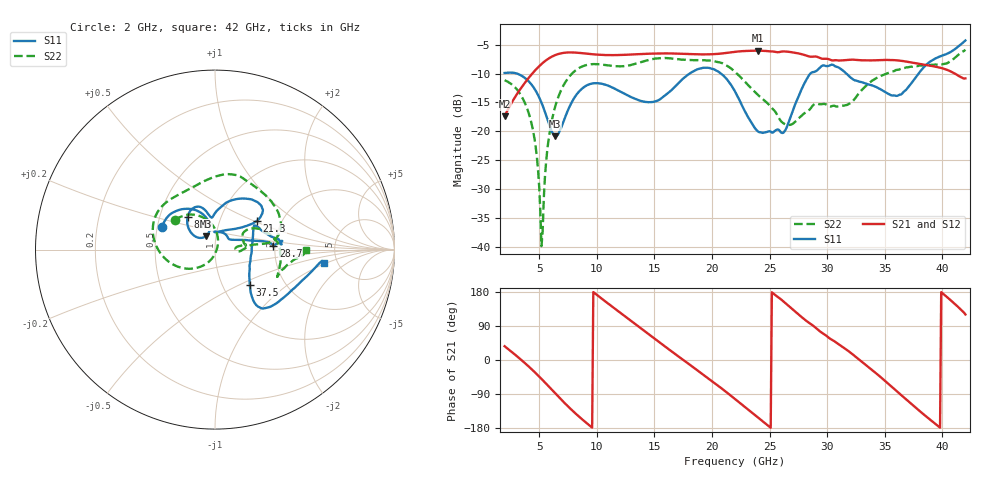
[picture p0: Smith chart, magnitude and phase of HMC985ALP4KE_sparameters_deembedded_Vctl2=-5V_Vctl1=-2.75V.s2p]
!s2p File: Measurements: S11, S21, S12, S22
# GHz S dB R 50.0
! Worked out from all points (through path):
!   401 points, 2 GHz to 42 GHz, reference 50 ohm
!   highest |S21| = -6.03 dB at 24 GHz (marker M1); lowest = -17.4 dB at 2 GHz (marker M2)
!   lowest |S11| = -20.9 dB at 6.4 GHz (marker M3), VSWR 1.20, Z = 44.7 + j6.77 ohm
!   |S11| at or under -10 dB: 3.095 GHz to 18.05 GHz (14.96 GHz wide, 141 % of centre); 20.79 GHz to 28.54 GHz (7.748 GHz wide, 31.4 % of centre); 31.67 GHz to 37.93 GHz (6.262 GHz wide, 18 % of centre)
!   |S22| runs from -39.9 to -5.9 dB; largest |S21 - S12| = 0.00055
!   S11 on the Smith chart (normalised r, x): 2 GHz: 0.53, +0.15; 8.8 GHz: 0.69, +0.27; 21.3 GHz: 1.50, +0.52; 28.7 GHz: 1.96, +0.10; 37.5 GHz: 1.34, -0.57; 42 GHz: 3.92, -0.95
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2  -9.89 157.1  -17.40 36.4  -17.41 36.4  -11.14 143.7
4.2  -11.57 121.0  -10.47 -20.1  -10.47 -20.1  -17.57 94.6
4.7  -12.97 111.9  -9.33 -34.6  -9.33 -34.6  -22.74 78.3
5.2  -15.03 104.5  -8.35 -49.8  -8.35 -49.8  -39.88 6.8
5.4  -16.06 102.8  -8.00 -56.0  -8.01 -56.0  -31.66 -92.8
5.8  -18.39 103.8  -7.41 -68.8  -7.42 -68.8  -21.68 -119.0
6.4  -20.86 123.9  -6.79 -88.1  -6.79 -88.1  -15.63 -140.1
8.7  -12.64 131.2  -6.45 -155.7  -6.46 -155.7  -8.79 162.5
8.8  -12.47 129.8  -6.48 -158.3  -6.48 -158.3  -8.71 160.7
12.5  -13.58 101.9  -6.74 114.3  -6.74 114.3  -8.68 110.7
15.4  -14.56 93.1  -6.52 47.7  -6.53 47.7  -7.34 77.3
18.1  -9.94 63.2  -6.61 -13.1  -6.61 -13.1  -7.64 55.8
21.3  -10.98 34.5  -6.40 -85.9  -6.40 -85.9  -8.64 14.4
22  -13.09 36.8  -6.22 -103.0  -6.22 -103.0  -9.69 8.9
24  -20.03 81.0  -6.03 -151.8  -6.03 -151.8  -13.69 7.5
26.3  -19.99 34.4  -6.16 151.8  -6.16 151.9  -18.71 -0.5
28.7  -9.76 3.9  -7.06 92.5  -7.07 92.5  -15.65 10.0
32.4  -11.16 23.8  -7.60 10.4  -7.60 10.4  -14.36 31.4
35.4  -13.59 7.6  -7.63 -65.1  -7.63 -65.0  -9.84 14.3
37.5  -11.15 -45.5  -8.11 -120.9  -8.11 -120.9  -8.78 -3.9
39.6  -7.20 -47.8  -8.87 -173.6  -8.88 -173.6  -8.46 -23.4
42  -4.26 -7.1  -10.82 120.1  -10.83 120.2  -5.87 -0.4
